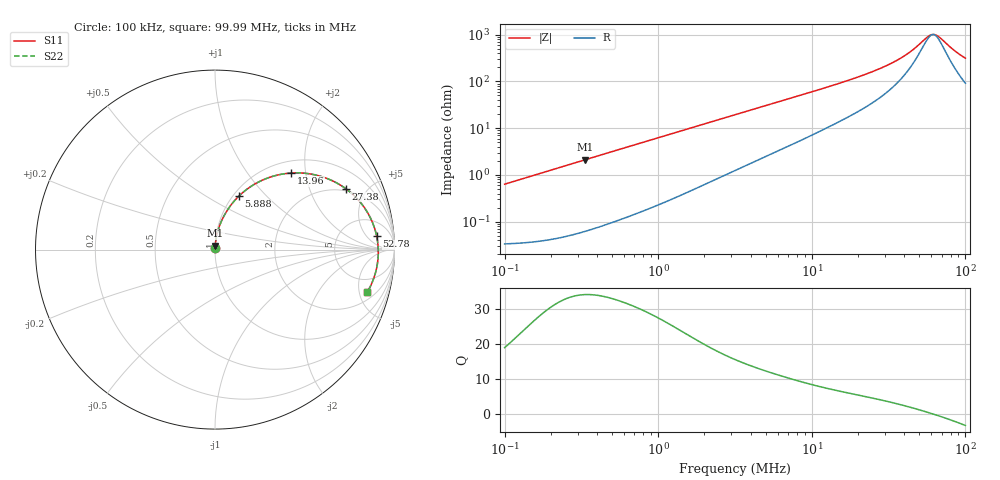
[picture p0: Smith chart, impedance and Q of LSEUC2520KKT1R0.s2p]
! LSEUC2520KKT1R0  S-PARAMETER MODEL  ( General Type )
! Model Generated by TAIYO YUDEN Corporation (http://www.ty-top.com)
! Version 1.0
! TAIYO YUDEN Control No. 220210
! Copyright(c) 2022 TAIYO YUDEN CO.,LTD. All Rights Reserved.
! Product Description (link to TY-COMPAS)
! https://ds.yuden.co.jp/TYCOMPAS/or/detail?pn=LSEUC2520KKT1R0M&u=M
! Products Name : Inductors
! Characteristics :
!  Inductance : 1.0 uH , SRF(min) : -Hz , DC Resistance(max) : 0.037 Ohm
!  Rated Current : Saturation :4400 mA , Temp Rise : 3600 mA (40 degC)
!  Case Size : 2.5 x 2.0 / 0.098 x 0.079 [mm/inch] , Thickness : 1 / 0.039 [mm/inch]
!  (Conditions: Temperature = 25 degC , DC Bias Current/Voltage = 0A / 0V)
! External Node Assignments :
!  1  o---GGG---o  2
! GND o---------o GND
! Frequency Range : 0.1MHz  -  99.992428MHz  [ 402 STEP ]
# MHz S RI R 50
! Freq[MHz].  S11 Real  S11 Imag  S21 Real  S21 Imag  S12 Real  S12 Imag  S22 Real  S22 Imag
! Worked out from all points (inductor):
!   401 points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, 100 kHz to 99.99 MHz, reference 50 ohm
!   read as one part in series: L = 1.01 uH near 103.5 kHz
!   highest Q = 34.1 at 335 kHz (marker M1), where L = 1 uH
!   self-resonance near 61.48 MHz
!   S11 on the Smith chart (normalised r, x): 100 kHz: 1.00, +0.01; 5.888 MHz: 1.06, +0.70; 13.96 MHz: 1.24, +1.66; 27.38 MHz: 1.87, +3.58; 52.78 MHz: 12, +10; 99.99 MHz: 2.83, -5.99
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0.1  0.000374 0.00632  0.9996 -0.00632  0.9996 -0.00632  0.000374 0.00632
0.318049  0.000993 0.0201  0.999 -0.0201  0.999 -0.0201  0.000993 0.0201
0.334961  0.00107 0.0211  0.9989 -0.0211  0.9989 -0.0211  0.00107 0.0211
1.011554  0.00624 0.0625  0.9938 -0.0625  0.9938 -0.0625  0.00624 0.0625
1.85134  0.0182 0.1116  0.9818 -0.1116  0.9818 -0.1116  0.0182 0.1116
3.162158  0.0467 0.1813  0.9533 -0.1813  0.9533 -0.1813  0.0467 0.1813
5.888173  0.1316 0.2967  0.8684 -0.2967  0.8684 -0.2967  0.1316 0.2967
7.762101  0.2006 0.3522  0.7994 -0.3522  0.7994 -0.3522  0.2006 0.3522
10.05722  0.2871 0.3965  0.7129 -0.3965  0.7129 -0.3965  0.2871 0.3965
13.96293  0.4236 0.4265  0.5764 -0.4265  0.5764 -0.4265  0.4236 0.4265
19.72309  0.5838 0.4097  0.4162 -0.4097  0.4162 -0.4097  0.5838 0.4097
27.38251  0.7278 0.3402  0.2722 -0.3402  0.2722 -0.3402  0.7278 0.3402
31.98693  0.7859 0.2901  0.2141 -0.2901  0.2141 -0.2901  0.7859 0.2901
41.44492  0.8608 0.1868  0.1392 -0.1868  0.1392 -0.1868  0.8608 0.1868
46.77036  0.8847 0.1323  0.1153 -0.1323  0.1153 -0.1323  0.8847 0.1323
52.78009  0.9008 0.0749  0.0992 -0.0749  0.0992 -0.0749  0.9008 0.0749
58.54228  0.9083 0.0242  0.0917 -0.0242  0.0917 -0.0242  0.9083 0.0242
61.65516  0.9097 -0.00144  0.0903 0.00144  0.0903 0.00144  0.9097 -0.00144
63.82183  0.9099 -0.0186  0.0901 0.0186  0.0901 0.0186  0.9099 -0.0186
68.38627  0.9081 -0.0531  0.0919 0.0531  0.0919 0.0531  0.9081 -0.0531
87.0899  0.88 -0.1723  0.12 0.1723  0.12 0.1723  0.88 -0.1723
99.99243  0.8485 -0.237  0.1515 0.237  0.1515 0.237  0.8485 -0.237
